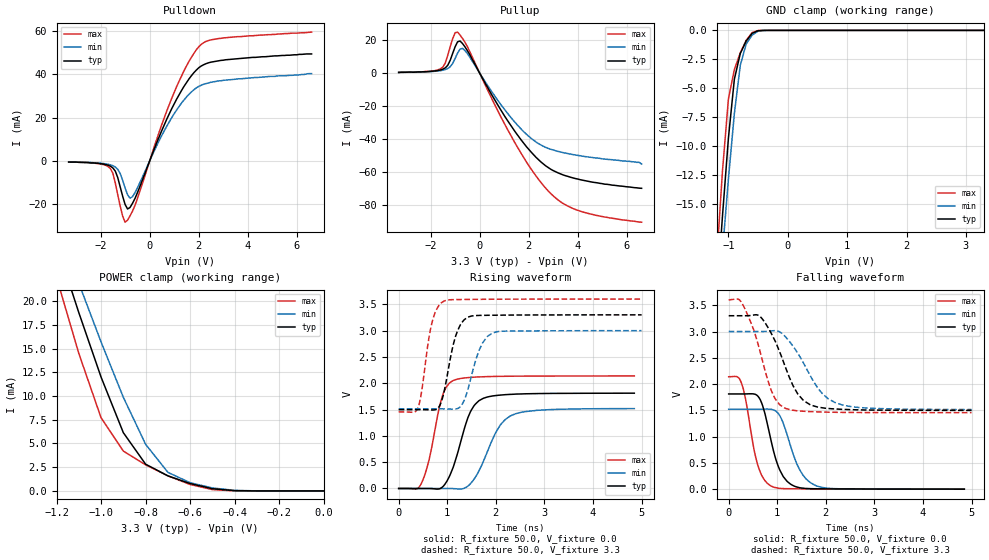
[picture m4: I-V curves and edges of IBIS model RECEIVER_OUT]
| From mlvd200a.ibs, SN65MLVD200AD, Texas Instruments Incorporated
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|   Receiver Output Model
[Model]   RECEIVER_OUT
Model_type   3-state
| Signals   R
Vmeas = 1.5V   |Reference voltage for timing measurements
Cref = 15pF   |Timing specification test load capacitance value
Vref = 0   |Timing specification test load voltage; GND
| variable   typ   min   max
C_comp   3.96pF   3.79pF   4.12pF
|   typ   min   max
[Temperature Range]   25.0   85   -40
[Voltage range]   3.3V   3.0V   3.6V
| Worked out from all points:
|   slope of the pulldown table from 0 to 0.495 V, typ, clamps not added: 35.2 ohm
|   slope of the pullup table from 0 to 0.495 V, typ, clamps not added: 37.6 ohm
|   GND clamp passes 1 mA (typ) near -0.71 V on its own axis
|   POWER clamp passes 1 mA (typ) near -0.63 V on its own axis
|   rising waveform, R_fixture 50.0, V_fixture 0.0: 20-80 % time 369ps typ, 465ps min, 293ps max; typ from 0 V to 1.81 V
|   falling waveform, R_fixture 50.0, V_fixture 0.0: 20-80 % time 310ps typ, 366ps min, 262ps max; typ from 1.81 V to 0.001 V
|   rising waveform, R_fixture 50.0, V_fixture 3.3: 20-80 % time 250ps typ, 292ps min, 212ps max; typ from 1.5 V to 3.3 V
|   falling waveform, R_fixture 50.0, V_fixture 3.3: 20-80 % time 502ps typ, 599ps min, 418ps max; typ from 3.3 V to 1.5 V
[Pulldown]
|   Voltage   I(typ)   I(min)   I(max)
-3.3V     -500uA     -400uA     -400uA
-1.6V     -2.42mA    -1.78mA    -3.49mA
-1.4V     -4.68mA    -2.79mA    -10.2mA
-1.2V     -12mA      -5.8mA     -20.9mA
-1V       -20.1mA    -12.5mA    -28.3mA
-900mV    -22.2mA    -15.6mA    -27.4mA
-700mV    -19.6mA    -16.5mA    -23.2mA
900mV     24.2mA     20mA       29mA
1.5V      36.2mA     29.6mA     43.9mA
2V        43.1mA     34.5mA     52.8mA
3V        46.6mA     37.3mA     56.9mA
6.6V      49.5mA     40.4mA     59.6mA
[Pullup]
|   Voltage   I(typ)   I(min)   I(max)
| Note that the[Pullup]voltage table is referenced to Vcc
| and is calculated using Vtable=Vcc - Vmeasured.
-3.3V     400uA      400uA      400uA
-1.6V     1.87mA     1.46mA     2.52mA
-1.3V     4.7mA      2.76mA     10.8mA
-1V       15.9mA     8.85mA     24.4mA
-900mV    18.9mA     12.1mA     24.8mA
-600mV    15.9mA     13.7mA     18.7mA
1.4V      -34.5mA    -29.1mA    -41.2mA
2.1V      -47.8mA    -39.5mA    -58.1mA
2.8V      -57.2mA    -45.6mA    -71.4mA
3.4V      -61.6mA    -48.1mA    -78.9mA
4.2V      -64.8mA    -50.3mA    -84mA
6.6V      -69.7mA    -55mA      -90.2mA
[GND_clamp]
|   Voltage   I(typ)   I(min)   I(max)
| Outputs in High Impedance (off)
-3.3V     -194mA     -176mA     -214mA
-1.2V     -23.4mA    -25.7mA    -20.1mA
-1.1V     -16.1mA    -19.2mA    -12.2mA
-1V       -9.35mA    -12.9mA    -5.95mA
-900mV    -4.24mA    -7.22mA    -3.4mA
-800mV    -2mA       -3.03mA    -1.95mA
-700mV    -915uA     -1.17mA    -851uA
-600mV    -249uA     -405uA     -194uA
-500mV    -29.2uA    -71.2uA    -13.4uA
-400mV    -1.66uA    -5.74uA    -320nA
3.3V      85.1pA     5.48uA     72.9pA
[POWER_clamp]
|   Voltage   I(typ)   I(min)   I(max)
| Note that the [POWER_clamp] voltage table is referenced to Vcc
| and is calculated using Vtable = Vcc - Vmeasured.
| Outputs in Tri-state.
-3.3V     190mA      172mA      209mA
-1.2V     26mA       28.3mA     22.5mA
-1.1V     18.8mA     21.9mA     14.5mA
-1V       12mA       15.7mA     7.71mA
-900mV    6.14mA     9.87mA     4.2mA
-800mV    2.82mA     4.92mA     2.75mA
-700mV    1.59mA     1.96mA     1.59mA
-600mV    776uA      867uA      677uA
-500mV    233uA      313uA      138uA
-400mV    27.2uA     58.6uA     7.1uA
0V        85.1pA     253pA      81.8pA
[Ramp]
|   typ   min   max
dV/dt_r   1.086V/368ps   0.912V/467ps   1.283V/293ps
dV/dt_f   1.084V/504ps   0.891V/599ps   1.287V/417ps
R_load = 50
[Rising Waveform]
R_fixture = 50.0
V_fixture = 0.0
V_fixture_min = 0.0
V_fixture_max = 0.0
C_fixture = 0p
L_fixture = 0n
|   V(typ)   V(min)   V(max)
0s        0V         0V         0V
475ps     0V         0V         112mV
625ps     0V         0V         540mV
900ps     27mV       0V         1.755V
1.125ns   410mV      -2mV       2.052V
1.475ns   1.454V     88mV       2.11V
1.75ns    1.716V     530mV      2.123V
2.075ns   1.773V     1.181V     2.131V
2.4ns     1.793V     1.418V     2.134V
4.85ns    1.811V     1.518V     2.138V
[Falling Waveform]
R_fixture = 50.0
V_fixture = 0.0
V_fixture_min = 0.0
V_fixture_max = 0.0
C_fixture = 0p
L_fixture = 0n
|   V(typ)   V(min)   V(max)
0s        1.812V     1.521V     2.139V
275ps     1.812V     1.521V     1.985V
600ps     1.772V     1.521V     457mV
700ps     1.586V     1.522V     231mV
875ps     914mV      1.52V      59mV
1.05ns    369mV      1.403V     17mV
1.2ns     152mV      1.044V     10mV
1.475ns   26mV       349mV      8mV
1.8ns     9mV        66mV       6mV
4.85ns    1mV        2mV        1mV
[Rising Waveform]
R_fixture = 50.0
V_fixture = 3.3
V_fixture_min = 3.0
V_fixture_max = 3.6
C_fixture = 0p
L_fixture = 0n
|   V(typ)   V(min)   V(max)
0s        1.498V     1.513V     1.455V
400ps     1.498V     1.513V     1.54V
700ps     1.491V     1.513V     3.204V
850ps     1.583V     1.513V     3.5V
950ps     1.906V     1.512V     3.567V
1.175ns   2.903V     1.51V      3.589V
1.425ns   3.255V     1.883V     3.592V
1.65ns    3.288V     2.614V     3.594V
1.925ns   3.292V     2.952V     3.596V
5ns       3.299V     2.999V     3.599V
[Falling Waveform]
R_fixture = 50.0
V_fixture = 3.3
V_fixture_min = 3.0
V_fixture_max = 3.6
C_fixture = 0p
L_fixture = 0n
|   V(typ)   V(min)   V(max)
0s        3.3V       3V         3.6V
275ps     3.3V       3V         3.535V
650ps     3.282V     2.999V     2.606V
875ps     2.967V     3.01V      1.882V
1.15ns    2.366V     2.917V     1.546V
1.325ns   1.969V     2.719V     1.502V
1.55ns    1.68V      2.382V     1.483V
1.925ns   1.549V     1.821V     1.468V
2.225ns   1.525V     1.634V     1.463V
5ns       1.499V     1.515V     1.456V
